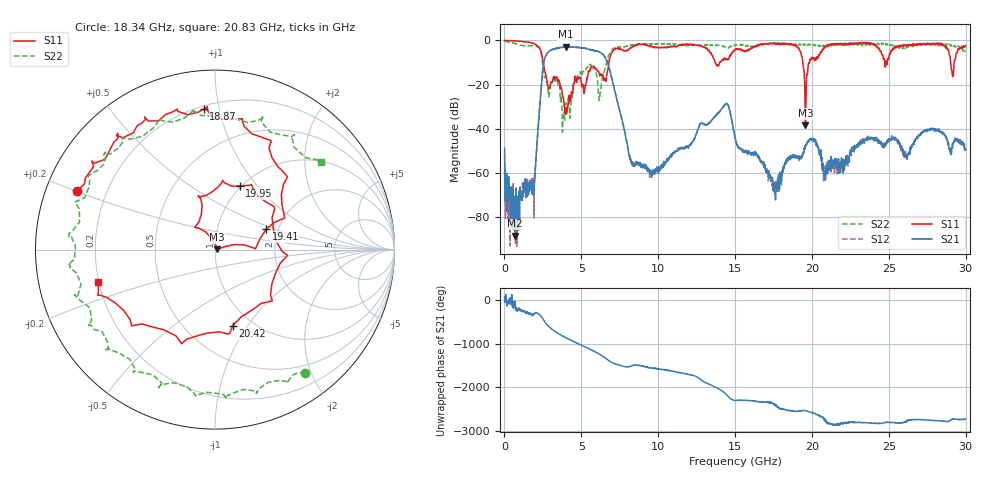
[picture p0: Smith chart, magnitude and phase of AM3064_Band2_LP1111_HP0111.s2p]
# Hz S DB R 50.0
!freq dBS11 angS11 dBS21 angS21 dBS12 angS12 dBS22 angS22
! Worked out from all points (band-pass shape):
!   1600 points, 10 MHz to 29.98 GHz, reference 50 ohm
!   highest |S21| = -2.89 dB at 4.002 GHz (marker M1); lowest = -88.4 dB at 703.5 MHz (marker M2)
!   |S21| within 3 dB of the highest: 2.773 GHz to 6.323 GHz (3.55 GHz wide, 78.1 % of centre)
!   lowest |S11| = -38.5 dB at 19.58 GHz (marker M3), VSWR 1.02, Z = 51.2 + j0.192 ohm
!   |S11| at or under -10 dB: 2.53 GHz to 6.788 GHz (4.258 GHz wide, 91.4 % of centre); 13.71 GHz to 13.99 GHz (277.4 MHz wide, 2 % of centre); 19.41 GHz to 19.83 GHz (425.9 MHz wide, 2.17 % of centre)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
!   |S22| runs from -41.6 to -0.1 dB; largest |S21 - S12| = 0.024
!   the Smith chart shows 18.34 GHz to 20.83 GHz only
!   S11 on the Smith chart (normalised r, x): 18.34 GHz: 0.09, +0.20; 18.87 GHz: 0.22, +0.90; 19.41 GHz: 1.73, +0.44; 19.95 GHz: 0.99, +0.82; 20.42 GHz: 0.82, -0.85; 20.83 GHz: 0.20, -0.13
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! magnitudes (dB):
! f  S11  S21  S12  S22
! 10 MHz  0.0  -48.8  -51.7  -0.1
! 703.5 MHz  -0.2  -88.4  -70.9  -1.4
! 1.903 GHz  -1.4  -64.3  -67.8  -2.4
! 2.672 GHz  -14.9  -7.2  -7.2  -16.2
! 4.002 GHz  -30.5  -2.9  -3.0  -29.0
! 5.015 GHz  -20.1  -3.4  -3.3  -15.4
! 6.627 GHz  -17.6  -8.8  -8.8  -10.2
! 8.313 GHz  -3.1  -55.4  -56.1  -2.1
! 10 GHz  -3.3  -58.4  -58.4  -1.6
! 14.37 GHz  -8.7  -28.7  -28.8  -3.2
! 15 GHz  -4.1  -44.5  -44.2  -2.2
! 17.61 GHz  -1.5  -68.3  -66.9  -1.0
! 18.34 GHz  -1.6  -55.3  -55.1  -1.4
! 18.87 GHz  -2.1  -52.4  -52.9  -2.2
! 19.41 GHz  -10.2  -51.9  -51.5  -1.7
! 19.58 GHz  -38.5  -48.2  -48.2  -2.1
! 19.95 GHz  -8.4  -44.4  -44.8  -2.1
! 19.99 GHz  -7.8  -44.7  -44.9  -1.7
! 20.42 GHz  -7.2  -48.8  -48.9  -2.6
! 20.83 GHz  -3.4  -62.6  -63.1  -2.3
! 25 GHz  -7.9  -45.9  -45.5  -1.5
! 29.98 GHz  -2.3  -49.4  -48.9  -4.4
